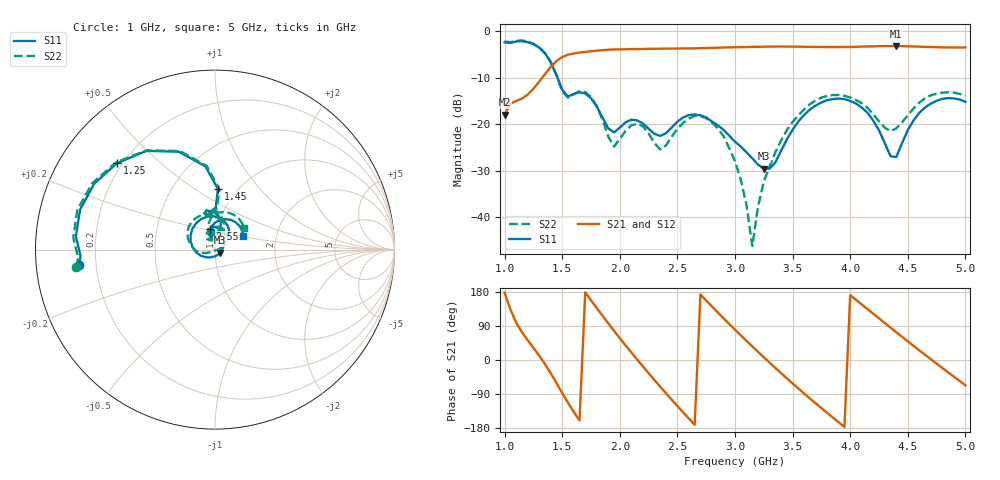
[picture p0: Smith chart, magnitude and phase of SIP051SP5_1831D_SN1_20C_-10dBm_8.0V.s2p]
# GHz  S  dB  R  50
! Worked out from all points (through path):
!   81 points, 1 GHz to 5 GHz, reference 50 ohm
!   highest |S21| = -3.16 dB at 4.4 GHz (marker M1); lowest = -18.0 dB at 1 GHz (marker M2)
!   lowest |S11| = -29.6 dB at 3.25 GHz (marker M3), VSWR 1.07, Z = 52.9 - j1.84 ohm
!   |S11| at or under -10 dB: 1.459 GHz to end of sweep
!   |S22| runs from -46.3 to -2.0 dB; largest |S21 - S12| = 0.003
!   S11 on the Smith chart (normalised r, x): 1 GHz: 0.14, -0.06; 1.25 GHz: 0.18, +0.37; 1.45 GHz: 0.82, +0.63; 2.55 GHz: 0.92, +0.22; 5 GHz: 1.35, +0.21
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1  -2.36 -173.4  -17.96 177.9  -17.95 177.7  -2.17 -172.8
1.25  -2.76 138.6  -12.38 32.1  -12.38 32.1  -2.67 138.5
1.45  -9.40 87.3  -6.40 -60.7  -6.40 -60.7  -9.47 85.8
1.55  -14.02 101.4  -5.03 -112.9  -5.03 -112.7  -14.30 101.3
1.7  -13.38 93.5  -4.44 178.6  -4.44 178.6  -13.08 92.0
1.85  -18.56 76.2  -4.04 116.7  -4.04 116.6  -19.04 65.3
1.95  -21.78 98.8  -3.89 76.9  -3.90 76.8  -24.84 96.9
2.15  -19.19 98.1  -3.81 1.4  -3.81 1.4  -19.94 99.9
2.35  -22.54 102.6  -3.74 -70.2  -3.74 -70.1  -25.45 103.7
2.55  -18.55 103.1  -3.67 -138.4  -3.69 -138.3  -19.73 115.6
2.75  -18.55 66.6  -3.59 156.9  -3.59 157.0  -18.71 74.5
3  -23.79 33.0  -3.42 80.0  -3.42 80.0  -28.02 21.4
3.15  -27.36 7.6  -3.34 35.8  -3.35 35.9  -46.30 -83.3
3.25  -29.60 -31.8  -3.30 7.2  -3.30 7.1  -32.39 -148.9
3.5  -21.20 -157.5  -3.29 -61.9  -3.29 -61.9  -19.53 -176.2
3.7  -15.99 148.9  -3.36 -114.3  -3.35 -114.3  -14.88 148.3
4  -15.00 82.0  -3.36 171.0  -3.36 171.1  -14.24 95.0
4.2  -19.24 46.1  -3.24 122.1  -3.22 122.2  -17.85 71.8
4.35  -26.92 59.8  -3.17 85.5  -3.17 85.4  -21.52 88.4
4.4  -27.09 90.7  -3.16 73.3  -3.17 73.4  -20.91 99.3
4.7  -15.56 80.7  -3.37 1.9  -3.37 2.0  -13.78 86.7
5  -15.17 25.7  -3.46 -66.9  -3.47 -66.8  -13.86 37.0
